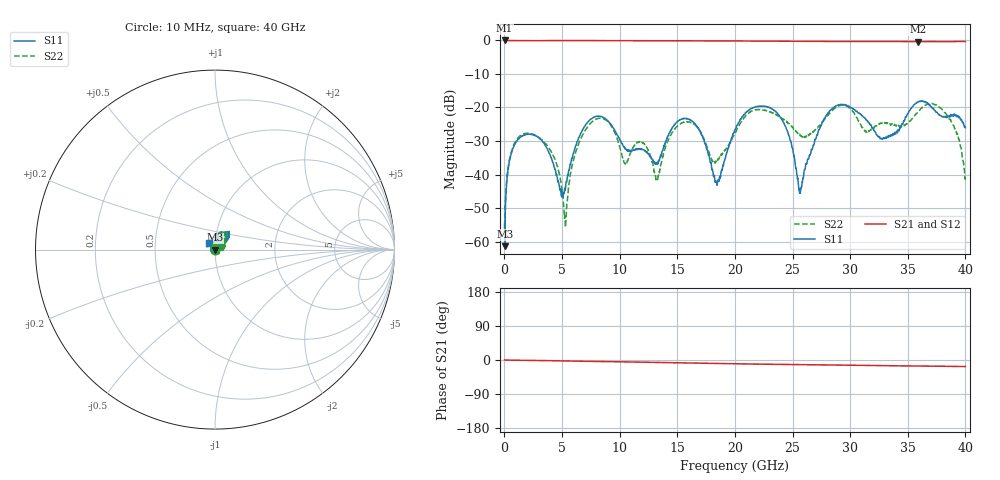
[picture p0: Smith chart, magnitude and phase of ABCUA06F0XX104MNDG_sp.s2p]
! Amotech Co.,Ltd.
! http://www.amotech.co.kr/
! Date: Thursday, December 03, 2020 09:49:36
! Part Number: ABCUA 06F 0XX 104M NDG
! Freq. Start=10[MHz] Stop=40[GHz], 4000[Steps]
# Hz S  dB  R 50
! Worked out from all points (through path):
!   4000 points, 10 MHz to 40 GHz, reference 50 ohm
!   highest |S21| = 0.00 dB at 10 MHz (marker M1); lowest = -0.4 dB at 35.86 GHz (marker M2)
!   group delay of S21, straight-line fit = 1.23 ps
!   lowest |S11| = -61.4 dB at 20 MHz (marker M3), VSWR 1.00, Z = 49.9 - j0.0403 ohm
!   |S11| at or under -10 dB: start of sweep to end of sweep
!   |S22| runs from -57.2 to -18.8 dB; largest |S21 - S12| = 0.0025
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1e7  -54.84 -116.5  0.00 0.1  -0.01 0.0  -54.08 -49.0
2e7  -61.38 -151.8  -0.00 0.0  -0.01 -0.0  -57.16 -3.7
4.4e8  -35.73 89.5  -0.02 -0.4  -0.02 -0.4  -35.38 74.8
1.21e9  -29.34 95.2  -0.06 -0.8  -0.06 -0.8  -28.95 68.9
3.89e9  -33.66 158.8  -0.04 -1.7  -0.03 -1.7  -32.22 18.5
5.28e9  -44.38 -29.9  -0.03 -2.4  -0.02 -2.4  -55.12 63.9
6.68e9  -27.35 49.7  -0.04 -3.2  -0.03 -3.2  -28.89 111.9
8.69e9  -23.19 74.0  -0.05 -4.1  -0.04 -4.1  -23.54 94.6
1.043e10  -32.06 141.5  -0.03 -4.9  -0.02 -5.0  -36.60 26.7
1.189e10  -32.54 -123.4  -0.04 -5.7  -0.03 -5.7  -30.21 -46.8
1.334e10  -36.00 -12.4  -0.05 -6.5  -0.04 -6.5  -40.61 38.8
1.594e10  -23.41 69.2  -0.07 -7.8  -0.07 -7.9  -24.26 79.4
1.845e10  -42.86 43.3  -0.10 -9.1  -0.09 -9.1  -36.11 10.0
2.001e10  -26.56 35.7  -0.14 -10.0  -0.13 -10.0  -27.58 48.4
2.349e10  -21.05 77.9  -0.22 -11.4  -0.22 -11.3  -21.95 55.2
2.567e10  -45.59 -1.7  -0.23 -12.2  -0.23 -12.2  -28.41 5.9
2.667e10  -32.66 -7.0  -0.25 -12.6  -0.25 -12.5  -27.50 -6.2
2.905e10  -19.13 43.9  -0.31 -13.5  -0.31 -13.5  -19.47 64.2
3.334e10  -28.80 10.1  -0.31 -15.1  -0.31 -15.2  -24.94 29.9
3.586e10  -18.35 49.6  -0.35 -15.9  -0.35 -16.0  -21.23 48.1
3.835e10  -22.98 77.5  -0.35 -16.6  -0.34 -16.7  -22.07 63.3
4e10  -26.04 133.4  -0.29 -17.3  -0.29 -17.3  -41.60 117.5
